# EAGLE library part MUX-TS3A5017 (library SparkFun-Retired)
Dual-channel 4:1 analog mux Retired: IC-08862
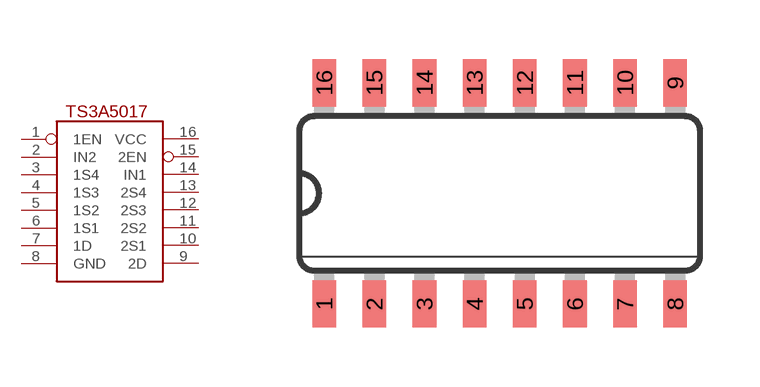
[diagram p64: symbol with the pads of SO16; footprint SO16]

Designator prefix -

## MUX-TS3A5017  [SO16]
1  1EN
2  IN2
3  1S4
4  1S3
5  1S2
6  1S1
7  1D
8  GND
9  2D
10  2S1
11  2S2
12  2S3
13  2S4
14  IN1
15  2EN
16  VCC

## Footprint SO16 (pad centres in mm)
Small Outline package 150 mil
smd 0.6 x 1.2: 1 -4.445,-2.8; 2 -3.175,-2.8; 3 -1.905,-2.8; 4 -0.635,-2.8; 5 0.635,-2.8; 6 1.905,-2.8; 7 3.175,-2.8; 8 4.445,-2.8; 9 4.445,2.8; 10 3.175,2.8; 11 1.905,2.8; 12 0.635,2.8; 13 -0.635,2.8; 14 -1.905,2.8; 15 -3.175,2.8; 16 -4.445,2.8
